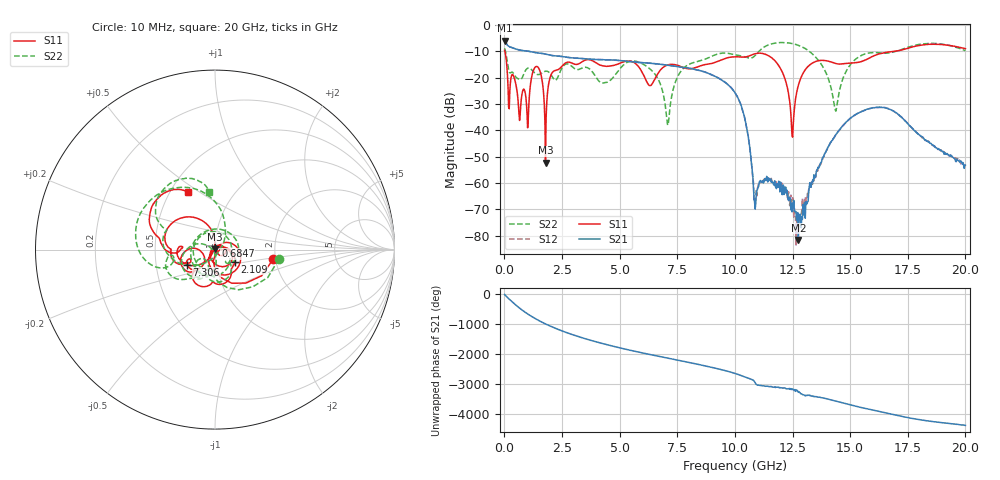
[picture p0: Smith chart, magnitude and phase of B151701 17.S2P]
!  2-Port S-parameters saved by WinCal
! VAR MeasName=S-Parameters (CALIBRATED_DATA) read from VNA (N5244A)
! VAR MeasDate=2015-12-24 19:10:08
! VAR NAME=B151701 17
! VAR FILENAME=B151701 17.S2P
! VAR DATE=2015-12-24 19:10:08
! VAR PHYS_PORTS=1,3
# Hz S DB R 50
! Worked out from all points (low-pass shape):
!   801 points, 10 MHz to 20 GHz, reference 50 ohm
!   highest |S21| = -5.95 dB at 10 MHz (marker M1); lowest = -81.6 dB at 12.75 GHz (marker M2)
!   |S21| within 3 dB of the highest: start of sweep to 421.3 MHz
!   lowest |S11| = -52.3 dB at 1.784 GHz (marker M3), VSWR 1.00, Z = 50 + j0.24 ohm
!   |S11| at or under -10 dB: 20.07 MHz to 16.96 GHz (16.94 GHz wide, 200 % of centre)
!   |S22| runs from -38.1 to -6.7 dB; largest |S21 - S12| = 0.0016
!   S11 on the Smith chart (normalised r, x): 10 MHz: 1.95, -0.23; 684.7 MHz: 1.00, +0.04; 2.109 GHz: 1.23, -0.17; 7.306 GHz: 0.72, -0.13; 20 GHz: 0.61, +0.45
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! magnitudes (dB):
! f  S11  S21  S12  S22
! 10 MHz  -9.6  -6.0  -5.9  -8.9
! 684.7 MHz  -34.0  -9.6  -9.6  -20.8
! 1.034 GHz  -35.7  -10.0  -10.0  -16.4
! 1.409 GHz  -15.8  -10.6  -10.6  -18.8
! 1.784 GHz  -52.3  -11.1  -11.1  -17.6
! 2.109 GHz  -17.8  -11.7  -11.7  -20.1
! 3.358 GHz  -14.1  -12.8  -12.8  -16.4
! 6.682 GHz  -18.2  -14.9  -14.9  -20.8
! 7.081 GHz  -15.2  -15.3  -15.3  -38.1
! 7.306 GHz  -15.0  -15.6  -15.6  -25.0
! 7.956 GHz  -16.6  -16.4  -16.4  -15.2
! 10.01 GHz  -12.1  -25.8  -25.7  -11.3
! 10.48 GHz  -12.2  -37.6  -37.6  -12.3
! 10.9 GHz  -10.9  -67.9  -64.9  -11.4
! 11.98 GHz  -16.6  -59.6  -59.9  -6.7
! 12.48 GHz  -41.7  -70.9  -67.7  -7.1
! 12.75 GHz  -22.9  -81.6  -72.8  -7.8
! 13.35 GHz  -14.5  -59.6  -60.5  -11.0
! 14.38 GHz  -14.6  -41.7  -41.7  -32.7
! 15.13 GHz  -14.4  -34.7  -34.7  -13.9
! 16.68 GHz  -10.3  -31.9  -31.8  -10.7
! 20 GHz  -9.0  -53.2  -53.3  -9.8
